TYPE MotionState_t :
 (
	MOTIONSTATE_INIT,
	MOTIONSTATE_ADJUSTCAMTABLE,
	MOTIONSTATE_ENABLE,
	MOTIONSTATE_COUPLE,
	MOTIONSTATE_MOVESLAVE,
	MOTIONSTATE_START,
	MOTIONSTATE_ERROR,
	MOTIONSTATE_RESET
 );
END_TYPE
